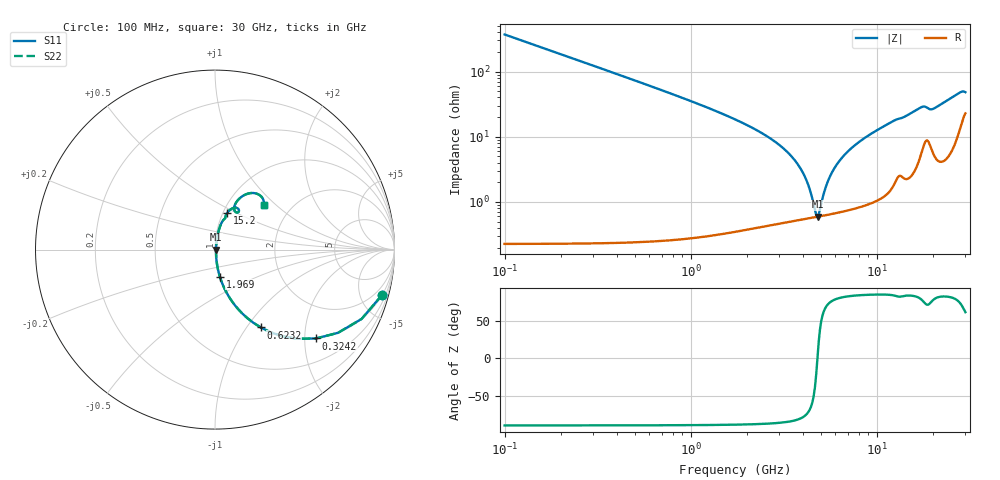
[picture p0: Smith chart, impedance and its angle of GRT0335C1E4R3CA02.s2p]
!Murata Part Number: GRT0335C1E4R3CA02
!These Parameters are Measured in Series Mode Connection
!Data Generated on Jun 19, 2026
!  o--ll--o
!Port1  Port2
!  o------o
!Operation Temp=25[degC], DC Bias Voltage=0[V]
!Freq. Start=100[MHz] Stop=30[GHz] 401[Steps]
# Hz S RI R 50
!Freq.(Hz) S11(Real) S11(Imag) S21(Real) S21(Imag) S12(Real) S12(Imag) S22(Real) S22(Imag)
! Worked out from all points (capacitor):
!   401 points, 100 MHz to 30 GHz, reference 50 ohm
!   read as one part in series: C = 4.3 pF near 249.5 MHz
!   lowest |Z| = 594 mohm at 4.809 GHz (marker M1)
!   series resonance near 4.806 GHz, so ESL is about 260 pH
!   S11 on the Smith chart (normalised r, x): 100 MHz: 1.00, -7.40; 324.2 MHz: 1.00, -2.27; 623.2 MHz: 1.00, -1.17; 1.969 GHz: 1.01, -0.31; 15.2 GHz: 1.05, +0.45; 30 GHz: 1.46, +0.85
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1e8  0.9318 -0.2518  0.0682 0.2518  0.0682 0.2518  0.9318 -0.2518
3.2425e8  0.5633 -0.495  0.4367 0.495  0.4367 0.495  0.5633 -0.495
6.2325e8  0.2548 -0.4336  0.7452 0.4336  0.7452 0.4336  0.2548 -0.4336
1.07175e9  0.0988 -0.2941  0.9012 0.2941  0.9012 0.2941  0.0988 -0.2941
1.96875e9  0.027 -0.1507  0.973 0.1507  0.973 0.1507  0.027 -0.1507
3.76275e9  0.0066 -0.0372  0.9934 0.0372  0.9934 0.0372  0.0066 -0.0372
4.21125e9  0.00591 -0.02  0.9941 0.02  0.9941 0.02  0.00591 -0.02
4.65975e9  0.00583 -0.00464  0.9942 0.00464  0.9942 0.00464  0.00583 -0.00464
4.80925e9  0.0059 0.000116  0.9941 -0.000116  0.9941 -0.000116  0.0059 0.000116
4.95875e9  0.00602 0.00473  0.994 -0.00473  0.994 -0.00473  0.00602 0.00473
5.10825e9  0.00618 0.00921  0.9938 -0.00921  0.9938 -0.00921  0.00618 0.00921
5.40725e9  0.0066 0.0178  0.9934 -0.0178  0.9934 -0.0178  0.0066 0.0178
5.70625e9  0.00716 0.026  0.9928 -0.026  0.9928 -0.026  0.00716 0.026
6.60325e9  0.00946 0.0486  0.9905 -0.0486  0.9905 -0.0486  0.00946 0.0486
8.0235e9  0.0147 0.0805  0.9853 -0.0805  0.9853 -0.0805  0.0147 0.0805
1.01165e10  0.0258 0.1225  0.9742 -0.1225  0.9742 -0.1225  0.0258 0.1225
1.505e10  0.0672 0.2029  0.9328 -0.2029  0.9328 -0.2029  0.0672 0.2029
1.51995e10  0.0691 0.2057  0.9309 -0.2057  0.9309 -0.2057  0.0691 0.2057
1.75915e10  0.12 0.2325  0.88 -0.2325  0.88 -0.2325  0.12 0.2325
2.005825e10  0.108 0.2198  0.892 -0.2198  0.892 -0.2198  0.108 0.2198
2.50665e10  0.1651 0.3047  0.8349 -0.3047  0.8349 -0.3047  0.1651 0.3047
3e10  0.2725 0.2511  0.7275 -0.2511  0.7275 -0.2511  0.2725 0.2511
